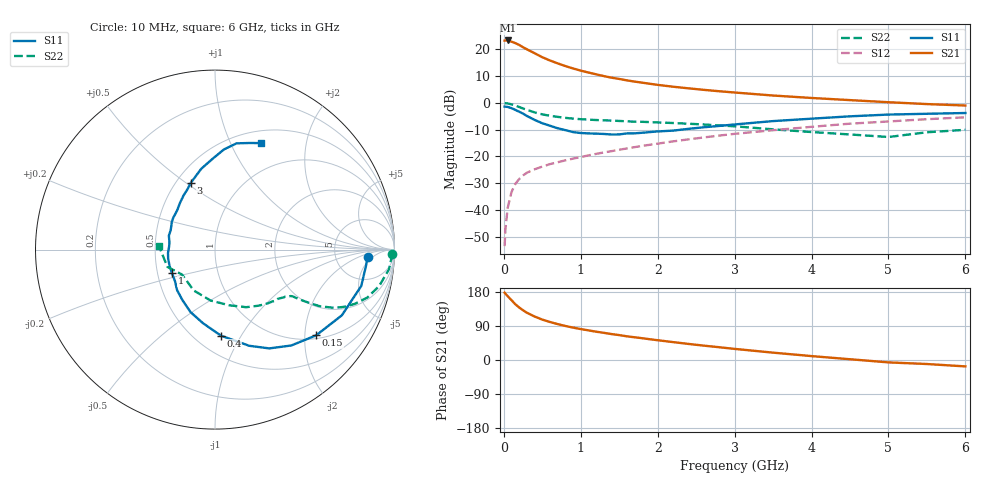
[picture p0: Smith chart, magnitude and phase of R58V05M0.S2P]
! SIEMENS Small Signal Semiconductors
! BFR183
! Si NPN RF Bipolar Junction Transistor in SOT23
! VCE = 8 V  IC = 5 mA
! Common Emitter S-Parameters:  May  1996
# GHz  S  MA  R  50
!  f  S11  S21  S12  S22
! GHz  MAG  ANG  MAG  ANG  MAG  ANG  MAG  ANG
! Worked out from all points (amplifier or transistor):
!   36 points, 10 MHz to 6 GHz, reference 50 ohm
!   highest |S21| = 23.3 dB at 50 MHz (marker M1)
!   |S21| within 3 dB of that: start of sweep to 280 MHz
!   unconditionally stable (mu >= 1): 1.095 GHz to 2.737 GHz
!   at 250 MHz: K = 0.41, MSG = 23.9 dB, |S12| = -27.1 dB
!   at 1.4 GHz: K = 1.06, MAG = 12.3 dB, |S12| = -18.0 dB
!   at 6 GHz: K = 0.87, MSG = 2.2 dB, |S12| = -5.4 dB
!   lowest NFmin = 1.15 dB at 450 MHz
!   S11 on the Smith chart (normalised r, x): 10 MHz: 11, -4; 150 MHz: 1.08, -2.28; 400 MHz: 0.66, -0.82; 1 GHz: 0.60, -0.17; 3 GHz: 0.59, +0.52; 6 GHz: 0.64, +1.31
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0.01  0.8512 -2.9  14.56 177.6  0.0021 86.9  0.9886 -1.3
0.02  0.8468 -5.8  14.63 174.9  0.0043 81.2  0.9847 -2.6
0.05  0.8396 -14.0  14.65 168.4  0.0109 83.4  0.9754 -6.5
0.1  0.7959 -27.4  13.89 157.8  0.0217 76.5  0.9369 -12.5
0.15  0.7388 -40.3  13.07 146.9  0.0307 70.0  0.8906 -17.4
0.2  0.6826 -51.5  12.08 138.5  0.0378 65.8  0.8359 -21.2
0.25  0.6282 -61.2  10.94 131.2  0.0441 62.0  0.7848 -24.0
0.3  0.5689 -70.4  10.01 124.6  0.0495 60.0  0.7407 -26.0
0.4  0.4803 -86.1  8.458 114.8  0.0574 57.5  0.6632 -28.4
0.5  0.4161 -99.1  7.116 106.6  0.0644 56.2  0.609 -29.4
0.6  0.3739 -111.4  6.187 100.3  0.0717 56.1  0.5742 -30.0
0.8  0.3092 -133.1  4.863 89.8  0.0843 56.2  0.5247 -30.8
1  0.2731 -151.6  4.001 81.6  0.0971 57.6  0.4953 -31.5
1.1  0.2689 -160.1  3.688 78.2  0.1044 58.2  0.486 -32.4
1.4  0.2562 176.1  2.955 68.4  0.1252 58.5  0.4664 -34.8
1.6  0.2685 163.2  2.631 62.5  0.1407 58.5  0.4514 -37.0
2.2  0.3029 134.3  2.002 47.2  0.1905 56.8  0.4202 -45.4
3  0.3949 110.1  1.561 29.3  0.2638 51.0  0.3648 -61.6
3.5  0.4565 99.7  1.371 19.4  0.3085 45.7  0.3201 -75.7
4.5  0.5602 84.9  1.125 2.0  0.4085 34.5  0.2567 -117.5
5.5  0.6253 71.8  0.949 -10.6  0.4955 22.4  0.2821 -160.0
6  0.6459 66.7  0.891 -16.9  0.5367 14.4  0.3136 176.1
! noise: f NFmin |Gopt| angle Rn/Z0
0.45  1.15  0.25  40  0.26
0.9  1.2  0.25  93  0.22
1.8  1.95  0.32  170  0.13
